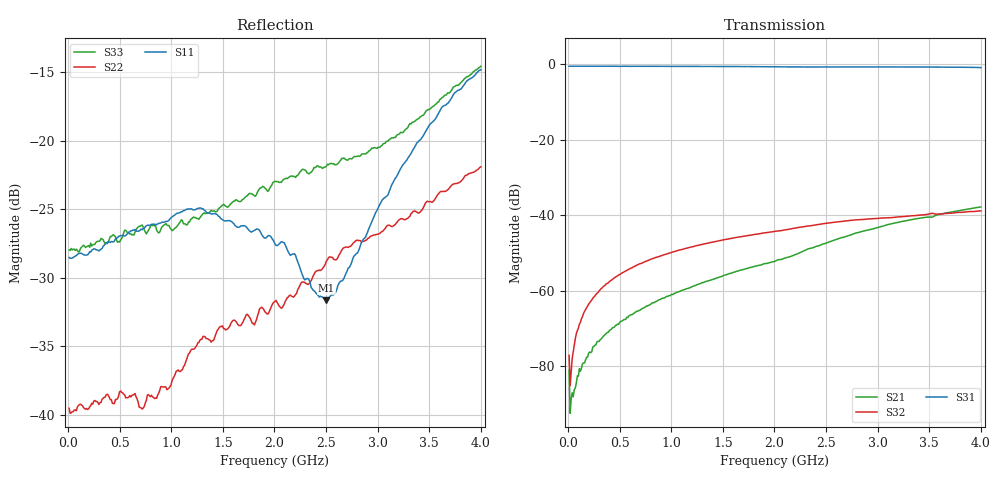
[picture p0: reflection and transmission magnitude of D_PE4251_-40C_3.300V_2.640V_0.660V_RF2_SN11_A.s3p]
! Device ID: PE4251_SoldCshunt_081809
! Dir: c:\Test Bench Repositories\Bench_Software_CVI_Version_8\trunk\PSC 4Port_VNA Bench\datalog\4250\TEST\PE4251_SoldCshunt_081809\-40C\3p300000\RF2
! Serial: 11
! Insertion: A
! Temp: -40C
! VDD: 3.300
! Control_Hi: 80.000
! Control_Lo: 20.000
! Logic State: RF2
! Port 1: RFC
! Port 2: RF1
! Port 3: RF2
! V1 = 0.66
! V2 = 0.66
! V3 = 0.66
! IDD: 4.418810e-05
! FILE NAME
! DATE 08/18/09  20:09
! CORRECTED  DATA
#  Hz  S  RI  R  50.00
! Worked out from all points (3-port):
!   401 points, 10 MHz to 4 GHz, reference 50 ohm
!   strongest paths, dB at 10 MHz, 1.008 GHz, 2.005 GHz, 3.002 GHz, 4 GHz:
!     S31: -0.5, -0.5, -0.6, -0.7, -0.9
!     S32: -77.2, -49.9, -44.3, -40.9, -38.9
!     S21: -81.2, -61.0, -52.2, -43.3, -37.8
!   lowest |S11| = -31.6 dB at 2.504 GHz (marker M1), VSWR 1.05, Z = 50.6 - j2.57 ohm
!   |S11| at or under -10 dB: start of sweep to end of sweep
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1e7  0.0375 -0.000717  4.67e-05 -4.7e-05  0.9448 -0.00329
     8.36e-05 -2.55e-05  0.0106 -0.000827  6.09e-05 2.03e-05
     0.9452 -0.00479  0.000138 1.28e-05  0.04 0.000763
3.9925e7  0.0373 0.000775  3.1e-05 -3.7e-05  0.9456 -0.0156
          2.12e-05 -3.87e-05  0.0103 -0.000111  2.84e-05 0.000126
          0.946 -0.0158  2.34e-05 0.000123  0.0399 0.0002
8.98e7  0.0384 0.00186  1.26e-05 -7.49e-05  0.9453 -0.0325
        1.88e-05 -7.14e-05  0.0107 0.000139  3.06e-05 0.000293
        0.9465 -0.0327  3.27e-05 0.000292  0.0398 -0.000654
1.696e8  0.0381 0.00323  -9.5e-06 -0.000122  0.9428 -0.0599
         -7.45e-06 -0.00012  0.0104 0.00137  4.57e-05 0.000563
         0.9438 -0.0601  4.38e-05 0.000557  0.0407 0.0016
4.78825e8  0.0439 0.00564  -0.000177 -0.000304  0.9277 -0.1659
           -0.000176 -0.000312  0.0111 0.00283  0.000146 0.00156
           0.9284 -0.1652  0.000145 0.00155  0.0425 -0.00259
7.18225e8  0.0473 0.00218  -0.0004 -0.000419  0.9101 -0.2441
           -0.000388 -0.000424  0.00986 0.00366  0.000275 0.00231
           0.9109 -0.2442  0.000267 0.0023  0.049 -0.00526
1.276825e9  0.0562 -0.00849  -0.0011 -0.000555  0.8393 -0.4188
            -0.0011 -0.000546  0.0169 0.00803  0.000695 0.00396
            0.8413 -0.4179  0.000703 0.00396  0.0516 -0.00888
2.005e9  0.0381 -0.0178  -0.00233 -0.000759  0.7028 -0.6057
         -0.00233 -0.000753  0.0164 0.0201  0.00126 0.00594
         0.7049 -0.6064  0.00125 0.00596  0.0653 -0.0282
2.50375e9  0.0065 -0.0254  -0.00409 -0.00125  0.5919 -0.7059
           -0.00408 -0.00126  0.0185 0.0314  0.00174 0.0076
           0.5948 -0.7053  0.00174 0.00762  0.053 -0.0608
4e9  -0.1798 -0.0223  -0.0127 0.00257  0.1397 -0.8972
     -0.0126 0.00256  -0.0299 0.0745  0.00286 0.011
     0.1408 -0.8953  0.00284 0.011  -0.1278 -0.1359
